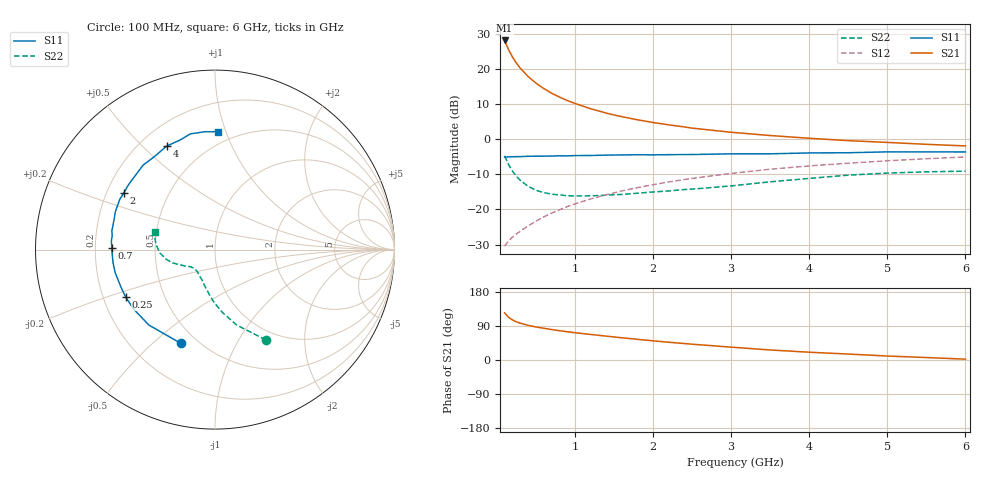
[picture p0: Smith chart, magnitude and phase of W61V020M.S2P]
! SIEMENS Small Signal Semiconductors
! BFR193W
! Si NPN RF Bipolar Junction Transistor in SOT323
! VCE = 1 V  IC = 20 mA
! Common Emitter S-Parameters:  September  1992
# GHz  S  MA  R  50
!  f  S11  S21  S12  S22
! GHz  MAG  ANG  MAG  ANG  MAG  ANG  MAG  ANG
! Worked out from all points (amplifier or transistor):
!   28 points, 100 MHz to 6 GHz, reference 50 ohm
!   highest |S21| = 28.1 dB at 100 MHz (marker M1)
!   |S21| within 3 dB of that: start of sweep to 160 MHz
!   unconditionally stable (mu >= 1): 661.6 MHz to 2.726 GHz
!   at 300 MHz: K = 0.78, MSG = 23.2 dB, |S12| = -26.2 dB
!   at 1.5 GHz: K = 1.05, MAG = 9.7 dB, |S12| = -15.3 dB
!   at 6 GHz: K = 0.95, MSG = 1.6 dB, |S12| = -5.1 dB
!   S11 on the Smith chart (normalised r, x): 100 MHz: 0.41, -0.62; 250 MHz: 0.29, -0.23; 700 MHz: 0.27, +0.01; 2 GHz: 0.27, +0.27; 4 GHz: 0.31, +0.59; 6 GHz: 0.41, +0.94
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0.1  0.5561 -109.9  25.27 124.3  0.0301 53.7  0.5778 -60.6
0.15  0.5588 -131.2  18.77 112.9  0.0358 51.3  0.4371 -74.0
0.2  0.5616 -143.7  14.76 105.7  0.0404 51.7  0.3532 -83.2
0.25  0.5637 -152.0  12.08 100.9  0.0448 52.9  0.2964 -90.7
0.3  0.564 -158.2  10.23 97.1  0.049 55.0  0.2605 -95.9
0.4  0.5707 -166.9  7.767 91.5  0.0583 58.5  0.2137 -105.0
0.5  0.5726 -172.4  6.269 87.3  0.068 61.0  0.1877 -111.9
0.6  0.5733 -177.3  5.255 83.7  0.0784 62.6  0.1741 -118.0
0.7  0.5751 178.9  4.509 80.4  0.0885 63.9  0.1652 -122.2
0.8  0.5795 175.3  3.972 77.4  0.0988 64.7  0.1612 -126.1
0.9  0.5778 172.4  3.542 74.7  0.1097 65.3  0.157 -129.1
1  0.5839 169.7  3.218 72.0  0.1201 65.4  0.1558 -131.6
1.2  0.5855 164.4  2.709 67.5  0.1411 65.3  0.1563 -137.1
1.5  0.5946 158.2  2.209 60.8  0.1723 64.5  0.1624 -142.1
2  0.5979 147.9  1.725 50.6  0.2253 61.8  0.1773 -148.1
2.2  0.6016 144.2  1.597 46.9  0.2459 60.4  0.1834 -149.7
3  0.6179 130.4  1.252 33.9  0.3255 54.0  0.2164 -157.1
3.5  0.6184 123.0  1.125 26.5  0.3734 49.5  0.2474 -162.6
4  0.6366 115.0  1.029 20.5  0.4162 44.9  0.2763 -168.6
4.5  0.6407 107.7  0.952 15.7  0.4544 40.6  0.3076 -176.5
5.5  0.6591 95.0  0.844 6.5  0.5262 31.7  0.3432 168.3
6  0.6572 88.6  0.801 2.2  0.5585 27.1  0.3505 163.7
